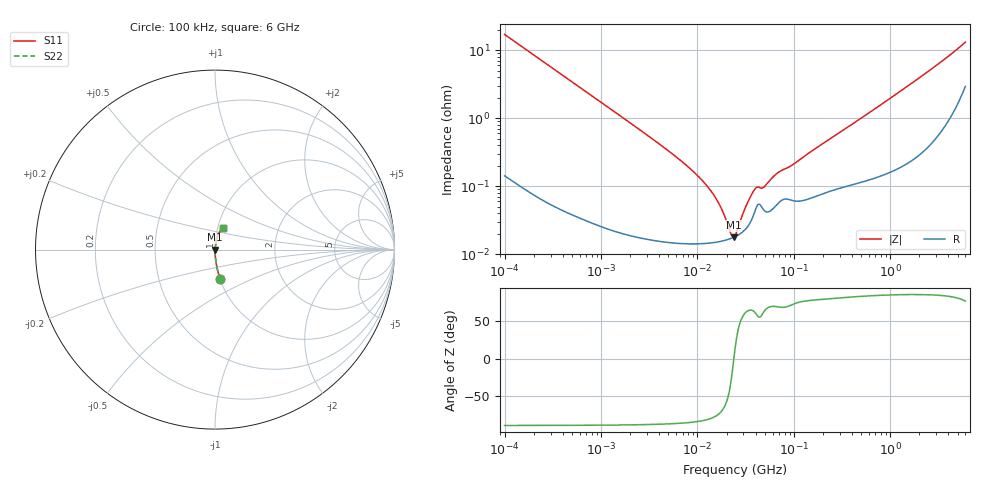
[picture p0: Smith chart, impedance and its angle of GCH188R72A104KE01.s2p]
!Murata Part Number: GCH188R72A104KE01
!These Parameters are Measured in Series Mode Connection
!Data Generated on Mar 13, 2026
!  o--ll--o
!Port1  Port2
!  o------o
!Operation Temp=25[degC], DC Bias Voltage=0[V]
!Freq. Start=100[kHz] Stop=6[GHz] 401[Steps]
# Hz S RI R 50
!Freq.(Hz) S11(Real) S11(Imag) S21(Real) S21(Imag) S12(Real) S12(Imag) S22(Real) S22(Imag)
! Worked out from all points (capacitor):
!   401 points, 100 kHz to 6 GHz, reference 50 ohm
!   read as one part in series: C = 93.7 nF near 105.7 kHz
!   lowest |Z| = 17.9 mohm at 23.83 MHz (marker M1)
!   series resonance near 23.84 MHz, so ESL is about 480 pH
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100000  0.0293 -0.1645  0.9707 0.1645  0.9707 0.1645  0.0293 -0.1645
228224  0.0062 -0.0741  0.9938 0.0741  0.9938 0.0741  0.0062 -0.0741
631452  0.00106 -0.027  0.9989 0.027  0.9989 0.027  0.00106 -0.027
3987316  0.000173 -0.00421  0.9998 0.00421  0.9998 0.00421  0.000173 -0.00421
8151931  0.000146 -0.00188  0.9999 0.00188  0.9999 0.00188  0.000146 -0.00188
1.265862e7  0.000146 -0.000988  0.9999 0.000988  0.9999 0.000988  0.000146 -0.000988
1.666634e7  0.000154 -0.000537  0.9998 0.000537  0.9998 0.000537  0.000154 -0.000537
1.860466e7  0.000159 -0.000369  0.9998 0.000369  0.9998 0.000369  0.000159 -0.000369
2.19429e7  0.00017 -0.000123  0.9998 0.000123  0.9998 0.000123  0.00017 -0.000123
2.318381e7  0.000176 -4.16e-05  0.9998 4.16e-05  0.9998 4.16e-05  0.000176 -4.16e-05
2.383034e7  0.000179 -6e-07  0.9998 6e-07  0.9998 6e-07  0.000179 -6e-07
2.517799e7  0.000185 8.18e-05  0.9998 -8.18e-05  0.9998 -8.18e-05  0.000185 8.18e-05
3.224998e7  0.000244 0.000474  0.9998 -0.000474  0.9998 -0.000474  0.000244 0.000474
3.700465e7  0.000339 0.000712  0.9997 -0.000712  0.9997 -0.000712  0.000339 0.000712
4.018763e7  0.000463 0.000817  0.9995 -0.000817  0.9995 -0.000817  0.000463 0.000817
4.872031e7  0.000447 0.000862  0.9996 -0.000862  0.9996 -0.000862  0.000447 0.000862
6.777267e7  0.000554 0.00147  0.9994 -0.00147  0.9994 -0.00147  0.000554 0.00147
9.690463e7  0.00062 0.00197  0.9994 -0.00197  0.9994 -0.00197  0.00062 0.00197
1.546735e8  0.00069 0.00325  0.9993 -0.00325  0.9993 -0.00325  0.00069 0.00325
9.76689e8  0.00195 0.0191  0.9981 -0.0191  0.9981 -0.0191  0.00195 0.0191
2.702311e9  0.0071 0.0527  0.9929 -0.0527  0.9929 -0.0527  0.0071 0.0527
6e9  0.0432 0.1185  0.9568 -0.1185  0.9568 -0.1185  0.0432 0.1185
